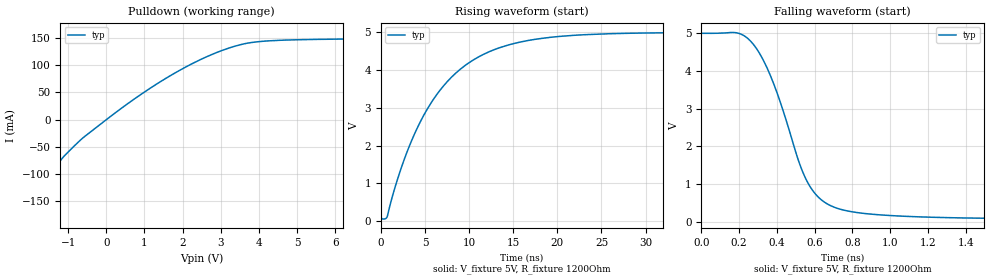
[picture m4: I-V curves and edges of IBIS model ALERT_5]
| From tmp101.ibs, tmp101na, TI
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|   ALERT 3.3V Model
[Model]   ALERT_5
Model_type   Open_drain
Polarity   Non-Inverting
Enable   Active-Low
Vmeas = 2.5
Vref = 2.5
Cref = 15pF
Rref = 1200
|   typ   min   max
C_comp   5.1566e-12   NA   NA
|C_comp (ON state)   1.000e-200   NA   NA
|C_comp (OFF state)   1.000e-200   NA   NA
[Voltage Range]   5   NA   NA
[Temperature Range]   27   NA   NA
[Pullup Reference]   5   NA   NA
[Pulldown Reference]   0   NA   NA
[Power Clamp Reference]   5   NA   NA
[GND Clamp Reference]   0   NA   NA
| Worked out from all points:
|   slope of the pulldown table from 0 to 0.75 V, typ, clamps not added: 19.3 ohm
|   falling waveform, V_fixture 5V, R_fixture 1200Ohm: 20-80 % time 208ps typ, NA min, NA max; typ from 5 V to 0.076 V
|   rising waveform, V_fixture 5V, R_fixture 1200Ohm: 20-80 % time 7.13ns typ, NA min, NA max; typ from 0.076 V to 5 V
[Pulldown]
|   Voltage   I(typ)   I(min)   I(max)
-5V       -626.9mA   NA         NA
-2.909V   -319.5mA   NA         NA
-1.685V   -139.8mA   NA         NA
-1.305V   -86.94mA   NA         NA
-1.122V   -68.19mA   NA         NA
-621.7mV  -33.98mA   NA         NA
237mV     12.65mA    NA         NA
1.811V    86.15mA    NA         NA
3.219V    131.6mA    NA         NA
4.237V    144.6mA    NA         NA
8.523V    152.6mA    NA         NA
9.985V    169.6mA    NA         NA
[Ramp]
R_load = 1200
|   typ   min   max
dV/dt_r   2.9541/7.13045e-009 NA   NA
dV/dt_f   2.95421/2.07728e-010 NA   NA
[Falling Waveform]
V_fixture = 5V
R_fixture = 1200Ohm
C_fixture = 0F
|   Time   V(typ)   V(min)   V(max)
0s        5V         NA         NA
199.3ps   4.996V     NA         NA
291.6ps   4.596V     NA         NA
384.6ps   3.638V     NA         NA
543.6ps   1.242V     NA         NA
586.7ps   850.5mV    NA         NA
639ps     570.2mV    NA         NA
833.5ps   242.2mV    NA         NA
1.309ns   113.1mV    NA         NA
47.25ns   76.14mV    NA         NA
[Rising Waveform]
V_fixture = 5V
R_fixture = 1200Ohm
C_fixture = 0F
|   Time   V(typ)   V(min)   V(max)
0s        76.14mV    NA         NA
703.6ps   111mV      NA         NA
1.665ns   944.7mV    NA         NA
2.892ns   1.789V     NA         NA
5.641ns   3.115V     NA         NA
8.608ns   3.947V     NA         NA
12.2ns    4.482V     NA         NA
16.64ns   4.785V     NA         NA
21.98ns   4.925V     NA         NA
47.25ns   5V         NA         NA
